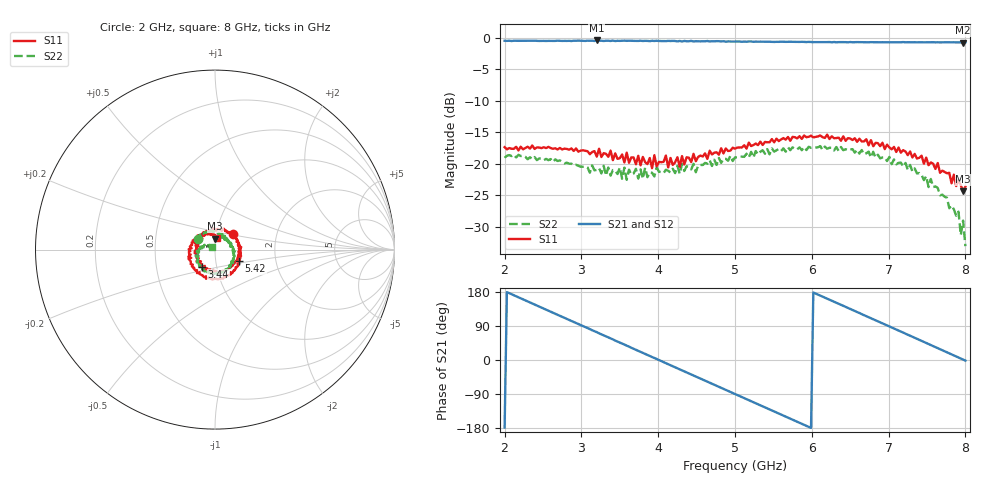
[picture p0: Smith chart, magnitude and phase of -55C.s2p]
!Agilent Technologies,E8361C,US49010292,A.09.42.06
!Agilent E8361C: A.09.42.06
!Date: Tuesday, January 14, 2025 01:37:32
!Correction: S11(Full 2 Port(1,2))
!S21(Full 2 Port(1,2))
!S12(Full 2 Port(1,2))
!S22(Full 2 Port(1,2))
!S2P File: Measurements: S11, S21, S12, S22:
# Hz S  dB  R 50
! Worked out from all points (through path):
!   201 points, 2 GHz to 8 GHz, reference 50 ohm
!   highest |S21| = -0.46 dB at 3.2 GHz (marker M1); lowest = -0.8 dB at 7.97 GHz (marker M2)
!   group delay of S21, straight-line fit = 251 ps
!   lowest |S11| = -24.4 dB at 7.97 GHz (marker M3), VSWR 1.13, Z = 49.7 + j6.03 ohm
!   |S11| at or under -10 dB: start of sweep to end of sweep
!   |S22| runs from -33.1 to -17.2 dB; largest |S21 - S12| = 0.011
!   S11 on the Smith chart (normalised r, x): 2 GHz: 1.21, +0.22; 3.44 GHz: 0.85, -0.17; 5.42 GHz: 1.30, -0.17; 8 GHz: 1.02, +0.13
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2e9  -17.37 40.9  -0.50 -178.3  -0.54 -178.0  -19.06 146.4
2.42e9  -17.41 -5.8  -0.53 143.7  -0.51 143.9  -19.43 117.3
2.72e9  -17.50 -42.2  -0.51 116.5  -0.54 116.4  -19.47 99.6
3.02e9  -17.86 -76.9  -0.53 89.6  -0.53 89.4  -20.47 82.0
3.2e9  -18.87 -94.0  -0.46 73.4  -0.55 73.1  -20.98 77.9
3.44e9  -18.35 -127.2  -0.55 51.2  -0.53 51.5  -21.10 55.5
3.77e9  -20.26 -171.4  -0.50 21.6  -0.59 21.5  -20.90 40.7
4.01e9  -19.70 155.8  -0.54 -0.2  -0.57 -0.3  -21.27 34.9
4.28e9  -20.48 116.7  -0.54 -24.8  -0.59 -24.7  -21.60 22.4
4.58e9  -18.86 77.7  -0.58 -51.9  -0.60 -51.9  -20.21 6.9
5e9  -17.61 25.4  -0.62 -89.8  -0.63 -89.7  -18.99 -19.5
5.42e9  -16.60 -24.9  -0.66 -127.7  -0.69 -127.7  -17.68 -49.5
5.72e9  -16.35 -55.6  -0.67 -155.0  -0.72 -154.8  -17.85 -68.2
6.02e9  -15.82 -87.6  -0.72 178.0  -0.74 178.0  -17.47 -89.0
6.29e9  -15.96 -116.5  -0.71 153.9  -0.75 153.7  -17.89 -106.9
6.59e9  -16.53 -145.8  -0.72 126.5  -0.75 126.8  -17.78 -131.7
7.01e9  -17.41 169.3  -0.76 88.6  -0.78 88.6  -18.91 -161.5
7.43e9  -18.73 124.4  -0.74 50.4  -0.77 50.6  -21.78 168.6
7.91e9  -22.57 88.2  -0.77 6.6  -0.77 6.7  -27.59 140.6
7.94e9  -23.41 83.3  -0.77 3.9  -0.78 3.8  -31.31 158.7
7.97e9  -24.37 89.0  -0.78 1.1  -0.78 1.1  -29.01 144.4
8e9  -23.63 78.7  -0.75 -1.6  -0.78 -1.7  -33.07 146.2
